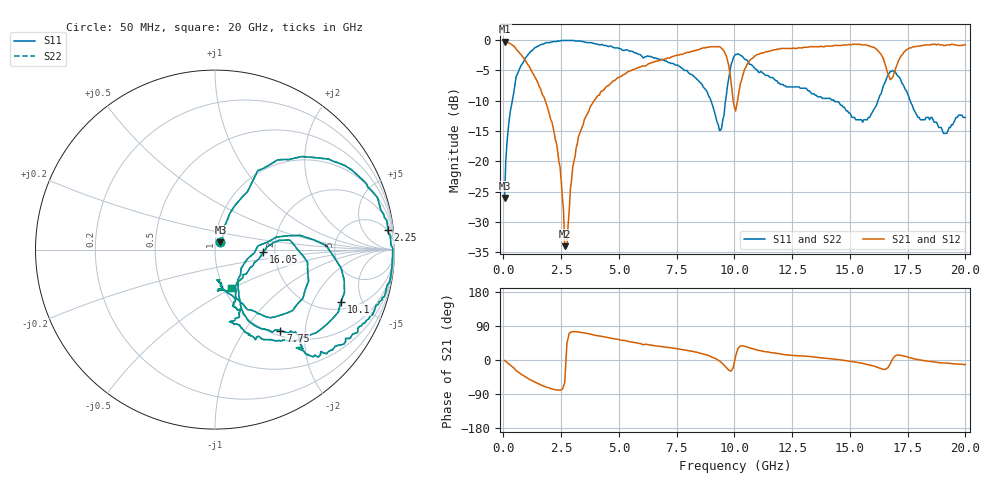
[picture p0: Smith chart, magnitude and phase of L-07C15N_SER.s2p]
#	mhz	s	ma	r	50
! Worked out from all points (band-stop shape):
!   400 points, 50 MHz to 20 GHz, reference 50 ohm
!   highest |S21| = -0.26 dB at 50 MHz (marker M1); lowest = -34.0 dB at 2.65 GHz (marker M2)
!   |S21| within 3 dB of the highest: 10.69 GHz to 16.46 GHz (5.771 GHz wide, 42.5 % of centre); 17.13 GHz to end of sweep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
!   lowest |S11| = -26.0 dB at 50 MHz (marker M3), VSWR 1.11, Z = 53 + j4.2 ohm
!   |S11| at or under -10 dB: 8.984 GHz to 9.617 GHz (633 MHz wide, 6.81 % of centre); 14.32 GHz to 16.22 GHz (1.897 GHz wide, 12.4 % of centre); 17.61 GHz to end of sweep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
!   |S22| runs from -26.0 to -0.1 dB; largest |S21 - S12| = 0
!   S11 on the Smith chart (normalised r, x): 50 MHz: 1.06, +0.08; 2.25 GHz: 5, +17; 7.75 GHz: 1.09, -1.48; 10.1 GHz: 2.42, -3.35; 16.05 GHz: 1.74, -0.05; 20 GHz: 1.09, -0.49
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50  0.05 52.3  0.97 -1.3  0.97 -1.3  0.05 52.3
200  0.18 67.6  0.95 -8.7  0.95 -8.7  0.18 67.6
550  0.5 61.6  0.84 -28.0  0.84 -28.0  0.5 61.6
1200  0.81 38.5  0.56 -53.3  0.56 -53.3  0.81 38.5
2250  0.97 6.4  0.15 -78.7  0.15 -78.7  0.97 6.4
2500  0.99 0.5  0.07 -78.5  0.07 -78.5  0.99 0.5
2650  0.99 -2.6  0.02 -61.2  0.02 -61.2  0.99 -2.6
3000  0.99 -9.6  0.09 74.6  0.09 74.6  0.99 -9.6
3400  0.97 -16.1  0.19 72.4  0.19 72.4  0.97 -16.1
6700  0.7 -46.9  0.67 36.5  0.67 36.5  0.7 -46.9
7750  0.58 -51.1  0.76 27.5  0.76 27.5  0.58 -51.1
9400  0.18 -25.4  0.87 -4.9  0.87 -4.9  0.18 -25.4
9750  0.48 9.5  0.62 -26.5  0.62 -26.5  0.48 9.5
10050  0.76 -18.4  0.26 9.7  0.26 9.7  0.76 -18.4
10100  0.76 -22.6  0.29 20.0  0.29 20.0  0.76 -22.6
11350  0.51 -68.6  0.8 21.6  0.8 21.6  0.51 -68.6
13350  0.36 -66.1  0.88 8.5  0.88 8.5  0.36 -66.1
16050  0.27 -2.6  0.87 -16.2  0.87 -16.2  0.27 -2.6
16700  0.53 -13.1  0.5 -14.7  0.5 -14.7  0.53 -13.1
17150  0.49 -50.8  0.7 12.7  0.7 12.7  0.49 -50.8
18050  0.22 -81.6  0.89 -0.2  0.89 -0.2  0.22 -81.6
20000  0.23 -66.8  0.91 -12.2  0.91 -12.2  0.23 -66.8
